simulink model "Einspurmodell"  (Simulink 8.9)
settings: Solver=ode1  StartTime=0.0  StopTime=SIM_time  FixedStep=1e-3  RelTol=1e-3  EnableMultiTasking=on
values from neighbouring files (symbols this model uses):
  Bf = 10.96    [parameter.m]
  Br = 12.67    [parameter.m]
  cf = 60000    [parameter.m]
  Cf = 1.1    [parameter.m]
  cr = 75000    [parameter.m]
  Cr = 1.3    [parameter.m]
  Fzeta0 = 8000    [parameter.m]
  Fzetaf = fzg_m*g*lh/l    (= 11216.8604651)    [parameter.m]
  Fzetar = fzg_m*g*(l-lh)/l    (= 6146.83953488)    [parameter.m]
  fzg_Jz = 1752    [parameter.m]
  fzg_m = 1770    [parameter.m]
  iL = 14    [parameter.m]
  k_Fzeta = 0.25    [parameter.m]
  lh = 1.75    [parameter.m]
  lv = (l-lh)    (= 0.959)    [parameter.m]
  manoever_choice = 1    [parameter.m]
  mu = 1.05    [parameter.m]
  speed = 10    [parameter.m]
  steering_angle = 30*pi/180    (= 0.523598775598)    [parameter.m]
  tire_choice = 1    [parameter.m]
undefined symbols (not defined in the file or in its folder): sinus_freq

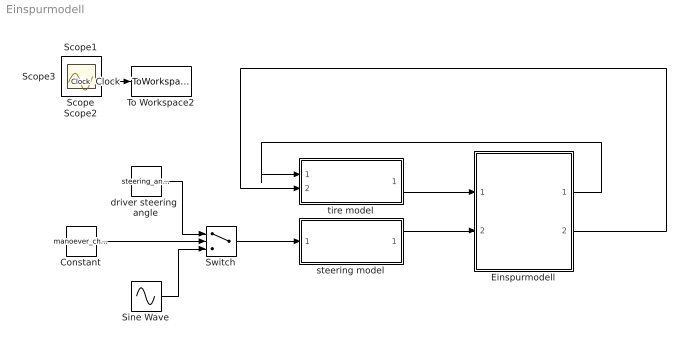
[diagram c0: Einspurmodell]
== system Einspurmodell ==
  Clock : Clock
  Constant : Constant  Value=manoever_choice
  Einspurmodell : Subsystem
  Sine Wave : Sin  Amplitude=steering_angle  Frequency=sinus_freq*2*pi  SampleTime=0
  Switch : Switch  Threshold=0.5
  To Workspace2 : ToWorkspace  VariableName=time  SampleTime=-1
  driver steering  angle : Constant  Value=steering_angle
  steering model : Subsystem
  tire model : Subsystem
  Scope{,1..3} (4 alike) : Scope
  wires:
  steering model/1(delta_r) -> Einspurmodell/2(delta_r)
  tire model/1(tire_info) -> Einspurmodell/1(Fy_tire)
  Einspurmodell/1(alpha_v) -> tire model/1(alpha_v)
  Clock/1 -> To Workspace2/1
  Switch/1 -> steering model/1(delta_lr)
  Constant/1 -> Switch/2
  driver steering  angle/1 -> Switch/1
  Sine Wave/1 -> Switch/3
  Einspurmodell/2(alpha_h) -> tire model/2(alpha_h)

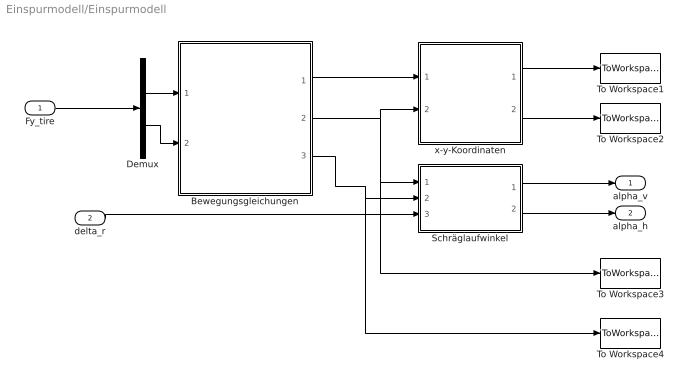
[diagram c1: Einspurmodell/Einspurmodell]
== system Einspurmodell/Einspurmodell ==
  Fy_tire : Inport
  delta_r : Inport  Port=2
  Bewegungsgleichungen : Subsystem
  Demux : Demux  Outputs=2
  Schräglaufwinkel : Subsystem
  To Workspace1 : ToWorkspace  VariableName=sim_x  SampleTime=-1
  To Workspace2 : ToWorkspace  VariableName=sim_y  SampleTime=-1
  To Workspace3 : ToWorkspace  VariableName=sim_beta  SampleTime=-1
  To Workspace4 : ToWorkspace  VariableName=sim_psip  SampleTime=-1
  x-y-Koordinaten : Subsystem
  alpha_v : Outport
  alpha_h : Outport  Port=2
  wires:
  Fy_tire/1 -> Demux/1
  Demux/1 -> Bewegungsgleichungen/1(Fyv)
  Demux/2 -> Bewegungsgleichungen/2(Fyh)
  delta_r/1 -> Schräglaufwinkel/3(delta_r)
  Bewegungsgleichungen/1(psi) -> x-y-Koordinaten/1(psi)
  Bewegungsgleichungen/2(beta) -> x-y-Koordinaten/2(beta), Schräglaufwinkel/1(beta), To Workspace3/1
  Schräglaufwinkel/1(alpha_v) -> alpha_v/1
  Bewegungsgleichungen/3(psi_p) -> Schräglaufwinkel/2(psi_p), To Workspace4/1
  x-y-Koordinaten/1(pos_x) -> To Workspace1/1
  x-y-Koordinaten/2(pos_y) -> To Workspace2/1
  Schräglaufwinkel/2(alpha_h) -> alpha_h/1

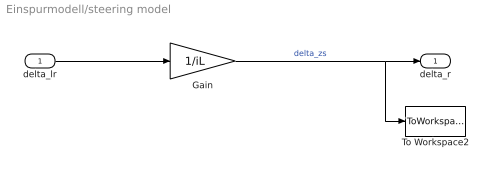
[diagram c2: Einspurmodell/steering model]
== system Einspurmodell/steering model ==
  delta_lr : Inport
  Gain : Gain  Gain=1/iL
  To Workspace2 : ToWorkspace  VariableName=sim_delta_r  SampleTime=-1
  delta_r : Outport
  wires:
  delta_lr/1 -> Gain/1
  Gain/1 -> To Workspace2/1, delta_r/1  "delta_zs"

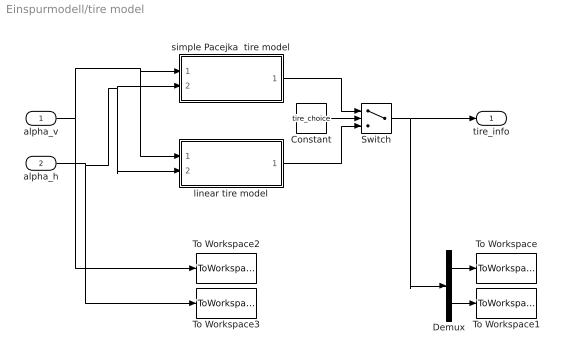
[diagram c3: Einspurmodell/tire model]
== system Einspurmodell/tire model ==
  alpha_v : Inport
  alpha_h : Inport  Port=2
  Constant : Constant  Value=tire_choice
  Demux : Demux  Outputs=2
  Switch : Switch  Threshold=0.5
  To Workspace : ToWorkspace  VariableName=sim_Fyf  SampleTime=-1
  To Workspace1 : ToWorkspace  VariableName=sim_Fyr  SampleTime=-1
  To Workspace2 : ToWorkspace  VariableName=sim_alphaf  SampleTime=-1
  To Workspace3 : ToWorkspace  VariableName=sim_alphar  SampleTime=-1
  linear tire model : MATLAB Function  TreatAsAtomicUnit=on
  simple Pacejka  tire model : MATLAB Function  TreatAsAtomicUnit=on
  tire_info : Outport
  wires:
  Constant/1 -> Switch/2
  simple Pacejka  tire model/1(Fy) -> Switch/1
  linear tire model/1(Fy) -> Switch/3
  Switch/1 -> tire_info/1, Demux/1
  Demux/1 -> To Workspace/1
  Demux/2 -> To Workspace1/1
  alpha_h/1 -> linear tire model/2(alpha_h), simple Pacejka  tire model/2(alpha_h), To Workspace3/1
  alpha_v/1 -> linear tire model/1(alpha_v), simple Pacejka  tire model/1(alpha_v), To Workspace2/1

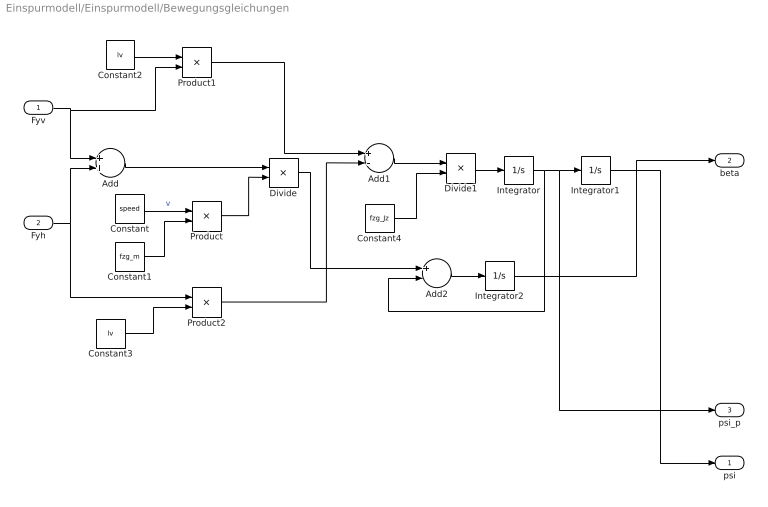
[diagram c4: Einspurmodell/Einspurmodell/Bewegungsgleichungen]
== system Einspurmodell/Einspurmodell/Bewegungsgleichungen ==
  Fyv : Inport
  Fyh : Inport  Port=2
  Add : Sum
  Add1 : Sum  Inputs=+-
  Add2 : Sum  Inputs=+-
  Constant : Constant  Value=speed
  Constant1 : Constant  Value=fzg_m
  Constant2 : Constant  Value=lv
  Constant3 : Constant  Value=lv
  Constant4 : Constant  Value=fzg_Jz
  Divide : Product  Inputs=*/
  Divide1 : Product  Inputs=*/
  Integrator : Integrator
  Integrator1 : Integrator
  Integrator2 : Integrator
  Product : Product
  Product1 : Product
  Product2 : Product
  psi : Outport
  beta : Outport  Port=2
  psi_p : Outport  Port=3
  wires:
  Fyh/1 -> Product2/1, Add/2
  Fyv/1 -> Product1/2, Add/1
  Constant/1 -> Product/1  "v"
  Constant1/1 -> Product/2
  Product/1 -> Divide/2
  Add/1 -> Divide/1
  Constant2/1 -> Product1/1
  Constant3/1 -> Product2/2
  Product1/1 -> Add1/1
  Product2/1 -> Add1/2
  Add1/1 -> Divide1/1
  Constant4/1 -> Divide1/2
  Divide1/1 -> Integrator/1
  Divide/1 -> Add2/1
  Integrator/1 -> psi_p/1, Integrator1/1, Add2/2
  Integrator1/1 -> psi/1
  Add2/1 -> Integrator2/1
  Integrator2/1 -> beta/1

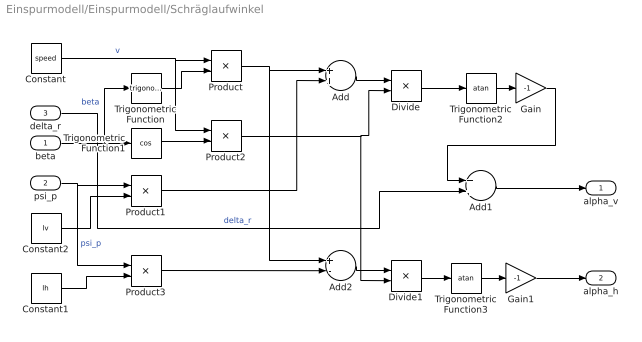
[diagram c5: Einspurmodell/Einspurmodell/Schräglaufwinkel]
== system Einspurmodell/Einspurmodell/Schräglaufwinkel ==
  beta : Inport
  psi_p : Inport  Port=2
  delta_r : Inport  Port=3
  Add : Sum
  Add1 : Sum
  Add2 : Sum  Inputs=+-
  Constant : Constant  Value=speed
  Constant1 : Constant  Value=lh
  Constant2 : Constant  Value=lv
  Divide : Product  Inputs=*/
  Divide1 : Product  Inputs=*/
  Gain : Gain  Gain=-1
  Gain1 : Gain  Gain=-1
  Product{,1..3} (4 alike) : Product
  Trigonometric Function : Trigonometry
  Trigonometric Function1 : Trigonometry  Operator=cos
  Trigonometric Function2 : Trigonometry  Operator=atan
  Trigonometric Function3 : Trigonometry  Operator=atan
  alpha_v : Outport
  alpha_h : Outport  Port=2
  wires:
  Constant/1 -> Product2/1, Product/1  "v"
  beta/1 -> Trigonometric Function1/1, Trigonometric Function/1  "beta"
  psi_p/1 -> Product3/1, Product1/1  "psi_p"
  Constant2/1 -> Product1/2
  Product1/1 -> Add/2
  Trigonometric Function/1 -> Product/2
  Product/1 -> Add2/1, Add/1
  Trigonometric Function1/1 -> Product2/2
  Add/1 -> Divide/1
  Product2/1 -> Divide1/2, Divide/2
  Divide/1 -> Trigonometric Function2/1
  Trigonometric Function2/1 -> Gain/1
  Gain/1 -> Add1/1
  delta_r/1 -> Add1/2  "delta_r"
  Constant1/1 -> Product3/2
  Product3/1 -> Add2/2
  Add1/1 -> alpha_v/1
  Add2/1 -> Divide1/1
  Divide1/1 -> Trigonometric Function3/1
  Trigonometric Function3/1 -> Gain1/1
  Gain1/1 -> alpha_h/1

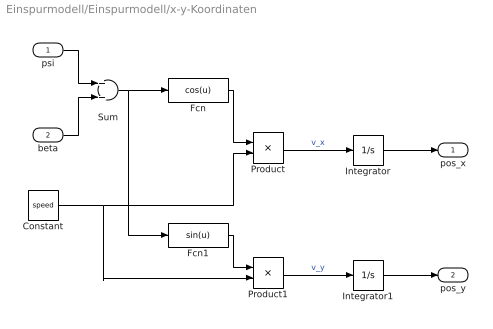
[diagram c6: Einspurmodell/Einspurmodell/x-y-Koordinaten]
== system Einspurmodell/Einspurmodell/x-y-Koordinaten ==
  psi : Inport
  beta : Inport  Port=2
  Constant : Constant  Value=speed
  Fcn : Fcn  Expr=cos(u)
  Fcn1 : Fcn  Expr=sin(u)
  Integrator : Integrator
  Integrator1 : Integrator
  Product : Product
  Product1 : Product
  Sum : Sum
  pos_x : Outport
  pos_y : Outport  Port=2
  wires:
  Constant/1 -> Product/2, Product1/2
  Fcn/1 -> Product/1
  Product/1 -> Integrator/1  "v_x"
  psi/1 -> Sum/1
  beta/1 -> Sum/2
  Sum/1 -> Fcn/1, Fcn1/1
  Fcn1/1 -> Product1/1
  Product1/1 -> Integrator1/1  "v_y"
  Integrator/1 -> pos_x/1
  Integrator1/1 -> pos_y/1

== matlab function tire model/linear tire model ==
function Fy = fcn(alpha_v, alpha_h, mu, cf, cr, Fzetaf, Fzetar)
%#eml

% slipf = alpha_info(1);
% slipr = alpha_info(2);
slipf = alpha_v;
slipr = alpha_h;

% Calculate Fmax:
Fmaxf = mu*Fzetaf;
Fmaxr = mu*Fzetar;

% Calculate slip curves
Fyf = mu * cf * slipf;
Fyr = mu * cr * slipr;

% % test on frition circle limit:(unzulässig, da sonst Probleme bei Schwimmwinkelberechnung)
% if abs(Fyf) > Fmaxf
%     Fyf = sign(Fyf)*Fmaxf;
% end
% 
% if abs(Fyr) > Fmaxr
%     Fyr = sign(Fyr)*Fmaxr;
% end

Fy = [Fyf; Fyr];

== matlab function tire model/simple Pacejka 
tire model ==
function Fy = fcn(alpha_v,alpha_h, mu, Cf, Cr, Bf, Br, Fzetaf, Fzetar, Fzeta0, k_Fzeta)
%#eml
slipf=alpha_v;
slipr=alpha_h;

Fmaxf=mu*Fzetaf*(1+(k_Fzeta*(Fzeta0-Fzetaf))/Fzeta0);
Fmaxr=mu*Fzetar*(1+(k_Fzeta*(Fzeta0-Fzetar))/Fzeta0);

Fyf=(Fmaxf*sin(Cf*atan(Bf*slipf/mu)));
Fyr=(Fmaxr*sin(Cr*atan(Br*slipr/mu)));

dummy = [Fyf; Fyr];


Fy = dummy;
